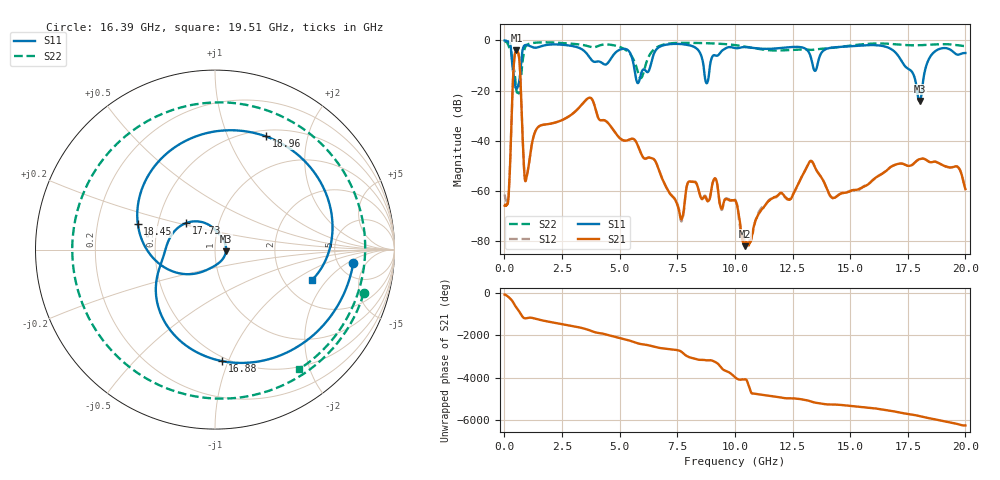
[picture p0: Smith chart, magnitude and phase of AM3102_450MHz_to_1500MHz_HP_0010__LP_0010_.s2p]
!Agilent Technologies,E8364B,MY43040894,A.07.50.67
!Agilent E8364B: A.07.50.67
!Date: Thursday, January 11, 2018 05:24:08
!Correction: S11(Full 2 Port(1,2))
!S21(Full 2 Port(1,2))
!S12(Full 2 Port(1,2))
!S22(Full 2 Port(1,2))
!S2P File: Measurements: S11, S21, S12, S22:
# Hz S  dB  R 50
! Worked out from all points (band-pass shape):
!   1601 points, 10 MHz to 20 GHz, reference 50 ohm
!   highest |S21| = -4.02 dB at 522.2 MHz (marker M1); lowest = -82.0 dB at 10.45 GHz (marker M2)
!   |S21| within 3 dB of the highest: 434.4 MHz to 639.7 MHz (205.3 MHz wide, 38.2 % of centre)
!   lowest |S11| = -24.2 dB at 18.01 GHz (marker M3), VSWR 1.13, Z = 56.5 - j1.2 ohm
!   |S11| at or under -10 dB: 347.8 MHz to 721.7 MHz (373.9 MHz wide, 69.9 % of centre); 5.613 GHz to 6.343 GHz (729.7 MHz wide, 12.2 % of centre); 17.35 GHz to 18.31 GHz (951.6 MHz wide, 5.34 % of centre)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
!   |S22| runs from -21.1 to -0.3 dB; largest |S21 - S12| = 0.00098
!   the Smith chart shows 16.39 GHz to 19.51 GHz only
!   S11 on the Smith chart (normalised r, x): 16.39 GHz: 6.90, -2.55; 16.88 GHz: 0.47, -0.95; 17.73 GHz: 0.69, +0.22; 18.45 GHz: 0.38, +0.14; 18.96 GHz: 0.57, +1.38; 19.51 GHz: 2.86, -1.41
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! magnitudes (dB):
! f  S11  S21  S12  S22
! 10 MHz  -0.1  -65.8  -61.3  -0.3
! 172.4 MHz  -0.6  -63.2  -62.8  -2.0
! 522.2 MHz  -18.7  -4.0  -4.0  -20.0
! 947 MHz  -1.9  -55.2  -55.2  -2.1
! 1.434 GHz  -2.8  -34.8  -34.8  -0.9
! 3.346 GHz  -3.5  -25.7  -25.7  -1.8
! 5.795 GHz  -17.0  -42.0  -42.0  -12.7
! 6.682 GHz  -2.9  -51.1  -51.0  -2.4
! 7.681 GHz  -1.5  -71.3  -72.2  -1.0
! 8.781 GHz  -17.1  -63.6  -63.0  -1.2
! 10.01 GHz  -3.1  -63.6  -63.5  -1.9
! 10.45 GHz  -2.7  -82.0  -80.4  -2.5
! 13.34 GHz  -8.4  -48.2  -48.2  -3.8
! 16.39 GHz  -2.2  -53.1  -53.1  -1.3
! 16.68 GHz  -3.0  -51.1  -51.0  -1.4
! 16.88 GHz  -4.1  -49.9  -49.8  -1.5
! 17.73 GHz  -13.2  -49.4  -49.3  -2.0
! 18.01 GHz  -24.2  -47.3  -47.3  -2.0
! 18.45 GHz  -6.9  -48.5  -48.5  -1.8
! 18.96 GHz  -3.2  -49.5  -49.5  -1.5
! 19.51 GHz  -4.9  -50.3  -50.2  -1.8
! 20 GHz  -5.1  -59.2  -58.8  -2.3
